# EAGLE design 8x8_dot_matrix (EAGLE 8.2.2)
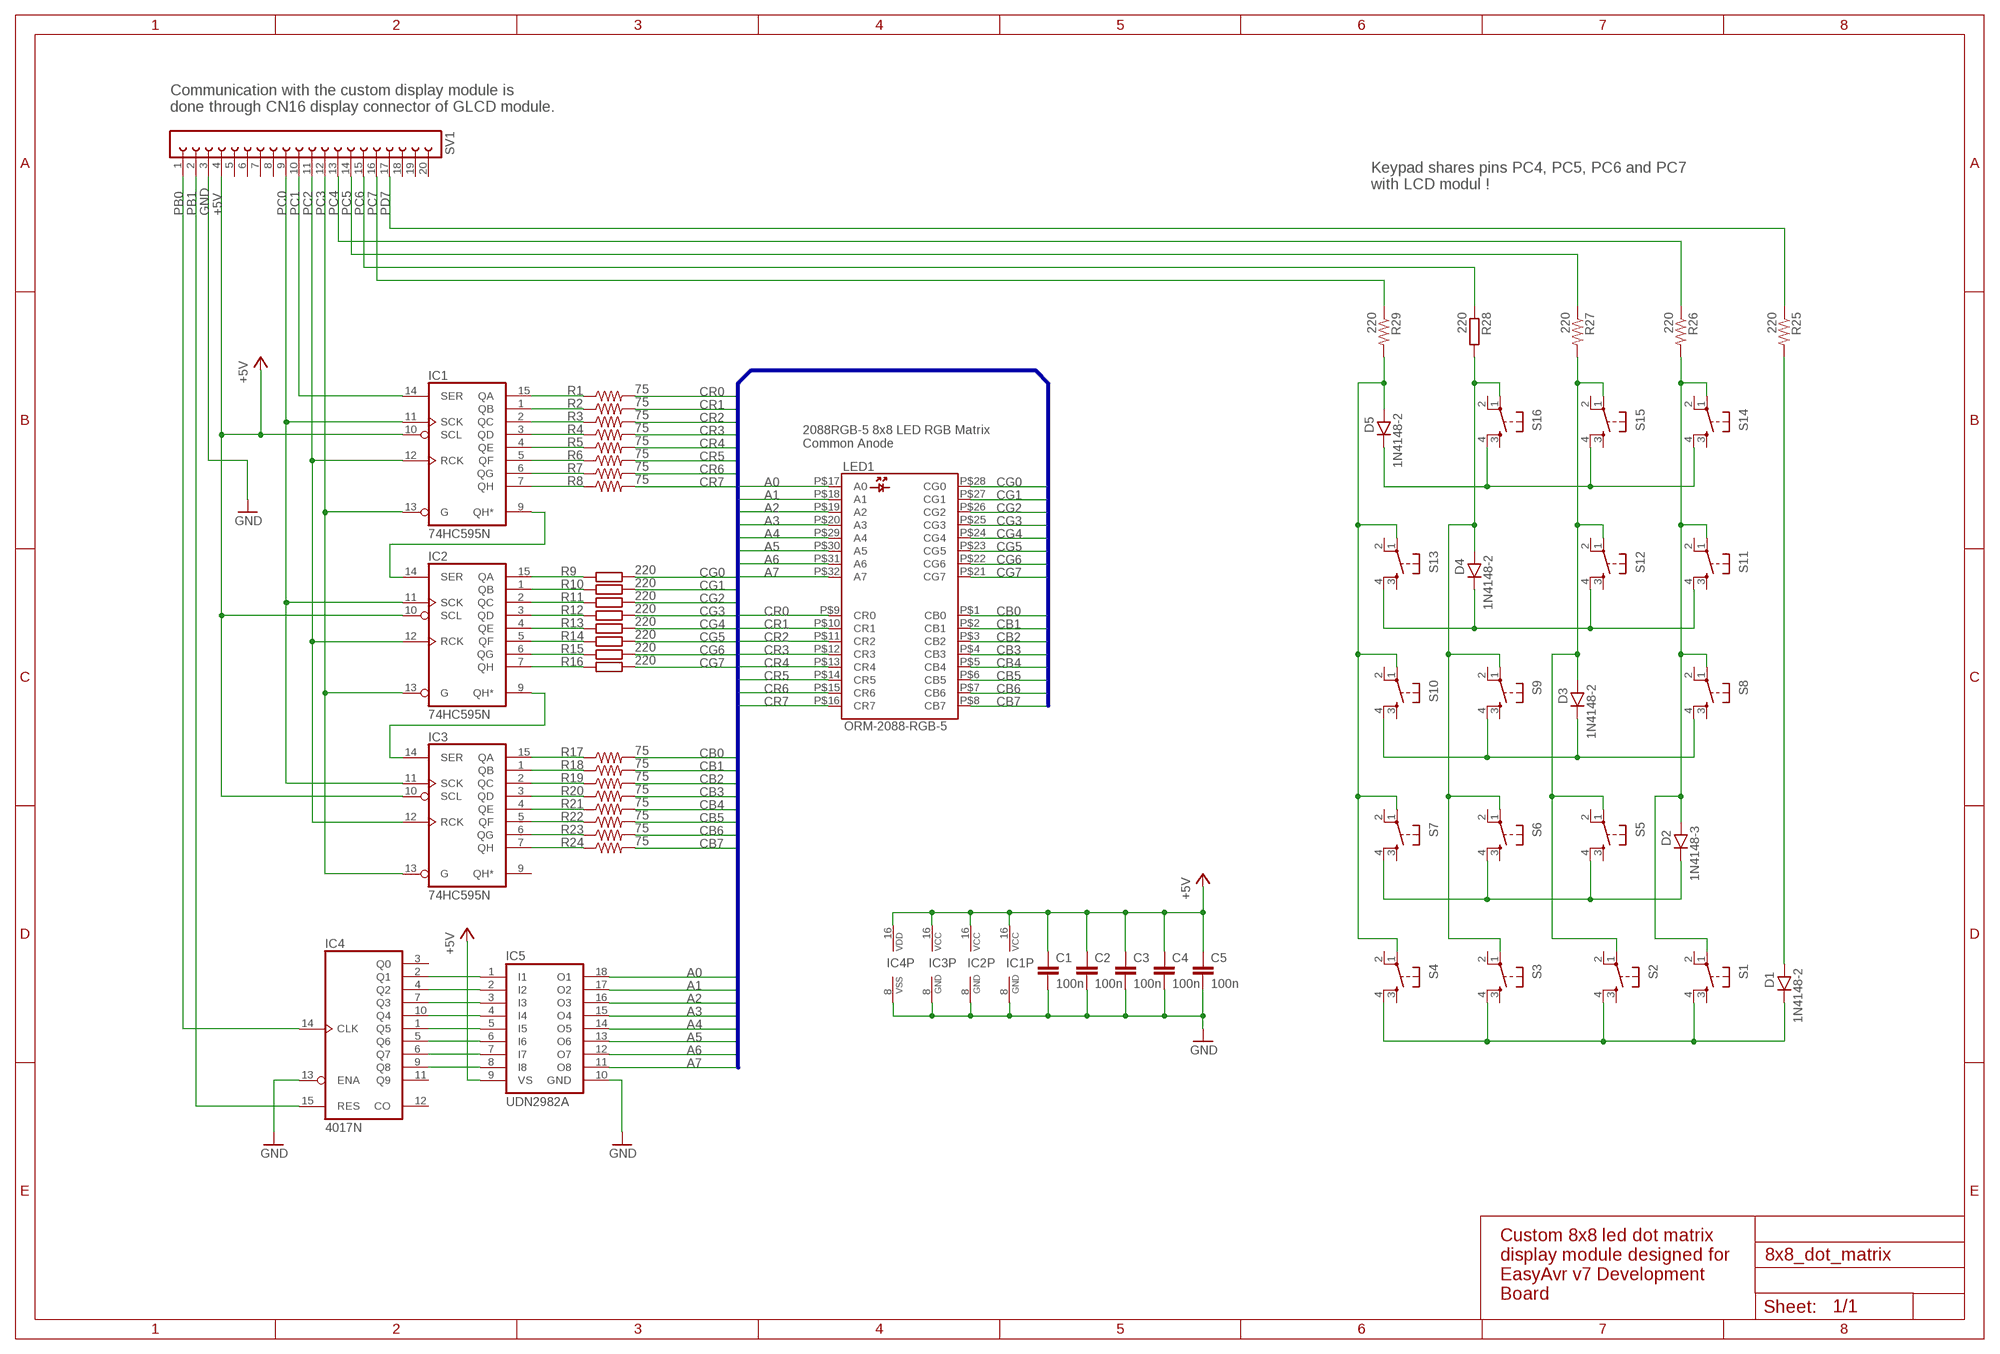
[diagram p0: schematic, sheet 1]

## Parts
C1  100n  C-EU050-024X044  [C050-024X044]
C2  100n  C-EU050-024X044  [C050-024X044]
C3  100n  C-EU050-024X044  [C050-024X044]
C4  100n  C-EU050-024X044  [C050-024X044]
C5  100n  C-EUC0805  [C0805]
D1  1N4148-2  [DO35-2]
D2  1N4148-3  [DO35-3]
D3  1N4148-2  [DO35-2]
D4  1N4148-2  [DO35-2]
D5  1N4148-2  [DO35-2]
IC1  74HC595N  [DIL16]
IC2  74HC595N  [DIL16]
IC3  74HC595N  [DIL16]
IC4  4017N  [DIL16]
IC5  UDN2982A  [DIL18]
LED1  ORM-2088-RGB-5  [ORM-2088-RGB-5]
R1  75  7MM  [0703]
R2  75  7MM  [0703]
R3  75  7MM  [0703]
R4  75  7MM  [0703]
R5  75  7MM  [0703]
R6  75  7MM  [0703]
R7  75  7MM  [0703]
R8  75  7MM  [0703]
R9  220  R-EU_0204/5  [0204/5]
R10  220  R-EU_0204/5  [0204/5]
R11  220  R-EU_0204/5  [0204/5]
R12  220  R-EU_0204/5  [0204/5]
R13  220  R-EU_0204/5  [0204/5]
R14  220  R-EU_0204/5  [0204/5]
R15  220  R-EU_0204/5  [0204/5]
R16  220  R-EU_0204/5  [0204/5]
R17  75  7MM  [0703]
R18  75  7MM  [0703]
R19  75  7MM  [0703]
R20  75  7MM  [0703]
R21  75  7MM  [0703]
R22  75  7MM  [0703]
R23  75  7MM  [0703]
R24  75  7MM  [0703]
R25  220  7MM  [0703]
R26  220  7MM  [0703]
R27  220  7MM  [0703]
R28  220  R-EU_0207/10  [0207/10]
R29  220  7MM  [0703]
S1  DTSM-6  [DTSM-6]
S2  DTSM-6  [DTSM-6]
S3  DTSM-6  [DTSM-6]
S4  DTSM-6  [DTSM-6]
S5  DTSM-6  [DTSM-6]
S6  DTSM-6  [DTSM-6]
S7  DTSM-6  [DTSM-6]
S8  DTSM-6  [DTSM-6]
S9  DTSM-6  [DTSM-6]
S10  DTSM-6  [DTSM-6]
S11  DTSM-6  [DTSM-6]
S12  DTSM-6  [DTSM-6]
S13  DTSM-6  [DTSM-6]
S14  DTSM-6  [DTSM-6]
S15  DTSM-6  [DTSM-6]
S16  DTSM-6  [DTSM-6]
SV1  FE20-1  [FE20]

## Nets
+5V: C1.1 C2.1 C3.1 C4.1 C5.1 IC1.10(SCL) IC1.16(VCC) IC2.10(SCL) IC2.16(VCC) IC3.10(SCL) IC3.16(VCC) IC4.16(VDD) IC5.9(VS) SV1.4
A0: IC5.18(O1) LED1.P$17(A0)
A1: IC5.17(O2) LED1.P$18(A1)
A2: IC5.16(O3) LED1.P$19(A2)
A3: IC5.15(O4) LED1.P$20(A3)
A4: IC5.14(O5) LED1.P$29(A4)
A5: IC5.13(O6) LED1.P$30(A5)
A6: IC5.12(O7) LED1.P$31(A6)
A7: IC5.11(O8) LED1.P$32(A7)
CB0: LED1.P$1(CB0) R17.2
CB1: LED1.P$2(CB1) R18.2
CB2: LED1.P$3(CB2) R19.2
CB3: LED1.P$4(CB3) R20.2
CB4: LED1.P$5(CB4) R21.2
CB5: LED1.P$6(CB5) R22.2
CB6: LED1.P$7(CB6) R23.2
CB7: LED1.P$8(CB7) R24.2
CG0: LED1.P$28(CG0) R9.2
CG1: LED1.P$27(CG1) R10.2
CG2: LED1.P$26(CG2) R11.2
CG3: LED1.P$25(CG3) R12.2
CG4: LED1.P$24(CG4) R13.2
CG5: LED1.P$23(CG5) R14.2
CG6: LED1.P$22(CG6) R15.2
CG7: LED1.P$21(CG7) R16.2
CR0: LED1.P$9(CR0) R1.2
CR1: LED1.P$10(CR1) R2.2
CR2: LED1.P$11(CR2) R3.2
CR3: LED1.P$12(CR3) R4.2
CR4: LED1.P$13(CR4) R5.2
CR5: LED1.P$14(CR5) R6.2
CR6: LED1.P$15(CR6) R7.2
CR7: LED1.P$16(CR7) R8.2
GND: C1.2 C2.2 C3.2 C4.2 C5.2 IC1.8(GND) IC2.8(GND) IC3.8(GND) IC4.8(VSS) IC4.13(ENA) IC5.10(GND) SV1.3
N$1: IC4.2(Q1) IC5.1(I1)
N$2: IC4.4(Q2) IC5.2(I2)
N$3: IC4.7(Q3) IC5.3(I3)
N$4: IC4.10(Q4) IC5.4(I4)
N$5: IC4.1(Q5) IC5.5(I5)
N$6: IC4.5(Q6) IC5.6(I6)
N$7: IC4.6(Q7) IC5.7(I7)
N$8: IC4.9(Q8) IC5.8(I8)
N$9: IC1.9(QH*) IC2.14(SER)
N$10: IC2.9(QH*) IC3.14(SER)
N$11: IC3.7(QH) R24.1
N$12: IC3.6(QG) R23.1
N$13: IC3.5(QF) R22.1
N$14: IC3.4(QE) R21.1
N$15: IC3.3(QD) R20.1
N$16: IC3.2(QC) R19.1
N$17: IC3.1(QB) R18.1
N$18: IC3.15(QA) R17.1
N$19: IC2.7(QH) R16.1
N$20: IC2.6(QG) R15.1
N$21: IC2.5(QF) R14.1
N$22: IC2.4(QE) R13.1
N$23: IC2.3(QD) R12.1
N$24: IC2.2(QC) R11.1
N$25: IC2.1(QB) R10.1
N$26: IC2.15(QA) R9.1
N$27: IC1.7(QH) R8.1
N$28: IC1.6(QG) R7.1
N$29: IC1.5(QF) R6.1
N$30: IC1.4(QE) R5.1
N$31: IC1.3(QD) R4.1
N$32: IC1.2(QC) R3.1
N$33: IC1.1(QB) R2.1
N$34: IC1.15(QA) R1.1
N$35: D2.C S5.4 S6.4 S7.4
N$36: D1.C S1.4 S2.4 S3.4 S4.4
N$37: D1.A R25.2
N$38: D3.C S8.4 S9.4 S10.4
N$39: D4.C S11.4 S12.4 S13.4
N$40: D5.C S14.4 S15.4 S16.4
N$41: D2.A R26.2 S1.1 S8.1 S11.1 S14.1
N$42: D3.A R27.2 S2.1 S5.1 S12.1 S15.1
N$43: D4.A R28.2 S3.1 S6.1 S9.1 S16.1
N$44: D5.A R29.2 S4.1 S7.1 S10.1 S13.1
PB0: IC4.14(CLK) SV1.1
PB1: IC4.15(RES) SV1.2
PC0: IC1.11(SCK) IC2.11(SCK) IC3.11(SCK) SV1.9
PC1: IC1.14(SER) SV1.10
PC2: IC1.12(RCK) IC2.12(RCK) IC3.12(RCK) SV1.11
PC3: IC1.13(G) IC2.13(G) IC3.13(G) SV1.12
PC4: R26.1 SV1.13
PC5: R27.1 SV1.14
PC6: R28.1 SV1.15
PC7: R29.1 SV1.16
PD7: R25.1 SV1.17
Unconnected: IC3.9(QH*) IC4.3(Q0) IC4.11(Q9) IC4.12(CO) S1.2 S1.3 S2.2 S2.3 S3.2 S3.3 S4.2 S4.3 S5.2 S5.3 S6.2 S6.3 S7.2 S7.3 S8.2 S8.3 S9.2 S9.3 S10.2 S10.3 S11.2 S11.3 S12.2 S12.3 S13.2 S13.3 S14.2 S14.3 S15.2 S15.3 S16.2 S16.3 SV1.5 SV1.6 SV1.7 SV1.8 SV1.18 SV1.19 SV1.20

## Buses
A[0..7],CR[0..7],CG[0..7],CB[0..7]

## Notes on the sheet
- Communication with the custom display module is
  done through CN16 display connector of GLCD module.
- Keypad shares pins PC4, PC5, PC6 and PC7
  with LCD modul !
- 2088RGB-5 8x8 LED RGB Matrix 
  Common Anode
- Custom 8x8 led dot matrix 
  display module designed for
  EasyAvr v7 Development
  Board

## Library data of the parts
C1-C5 = rcl:C-EU: CAPACITOR, European symbol
D1-D5 = gm-diodes:1N4148: Fast Switching Diode
IC1-IC3 = 74xx-eu:74*595: 8-bit SHIFT REGISTER, output latch
IC4 = 40xx:4017: COUNTER/DIVIDER
IC5 = uln-udn:UDN298*: DRIVER ARRAY Source: Allegro Microsystems Inc. / UDN2981-UDN2984.pdf
LED1 = LED:ORM-2088-RGB-5: ORM 2088RGB-5 8x8 LED RGB Matrix
R1-R8 R17-R27 R29 = gm-resistors:7MM: 7mm Resistors
R9-R16 R28 = rcl:R-EU_: RESISTOR, European symbol
S1-S16 = switch-tact:DTSM-6
SV1 = con-lsta:FE20-1: FEMALE HEADER; OC_FARNELL: unknown; OC_NEWARK: unknown

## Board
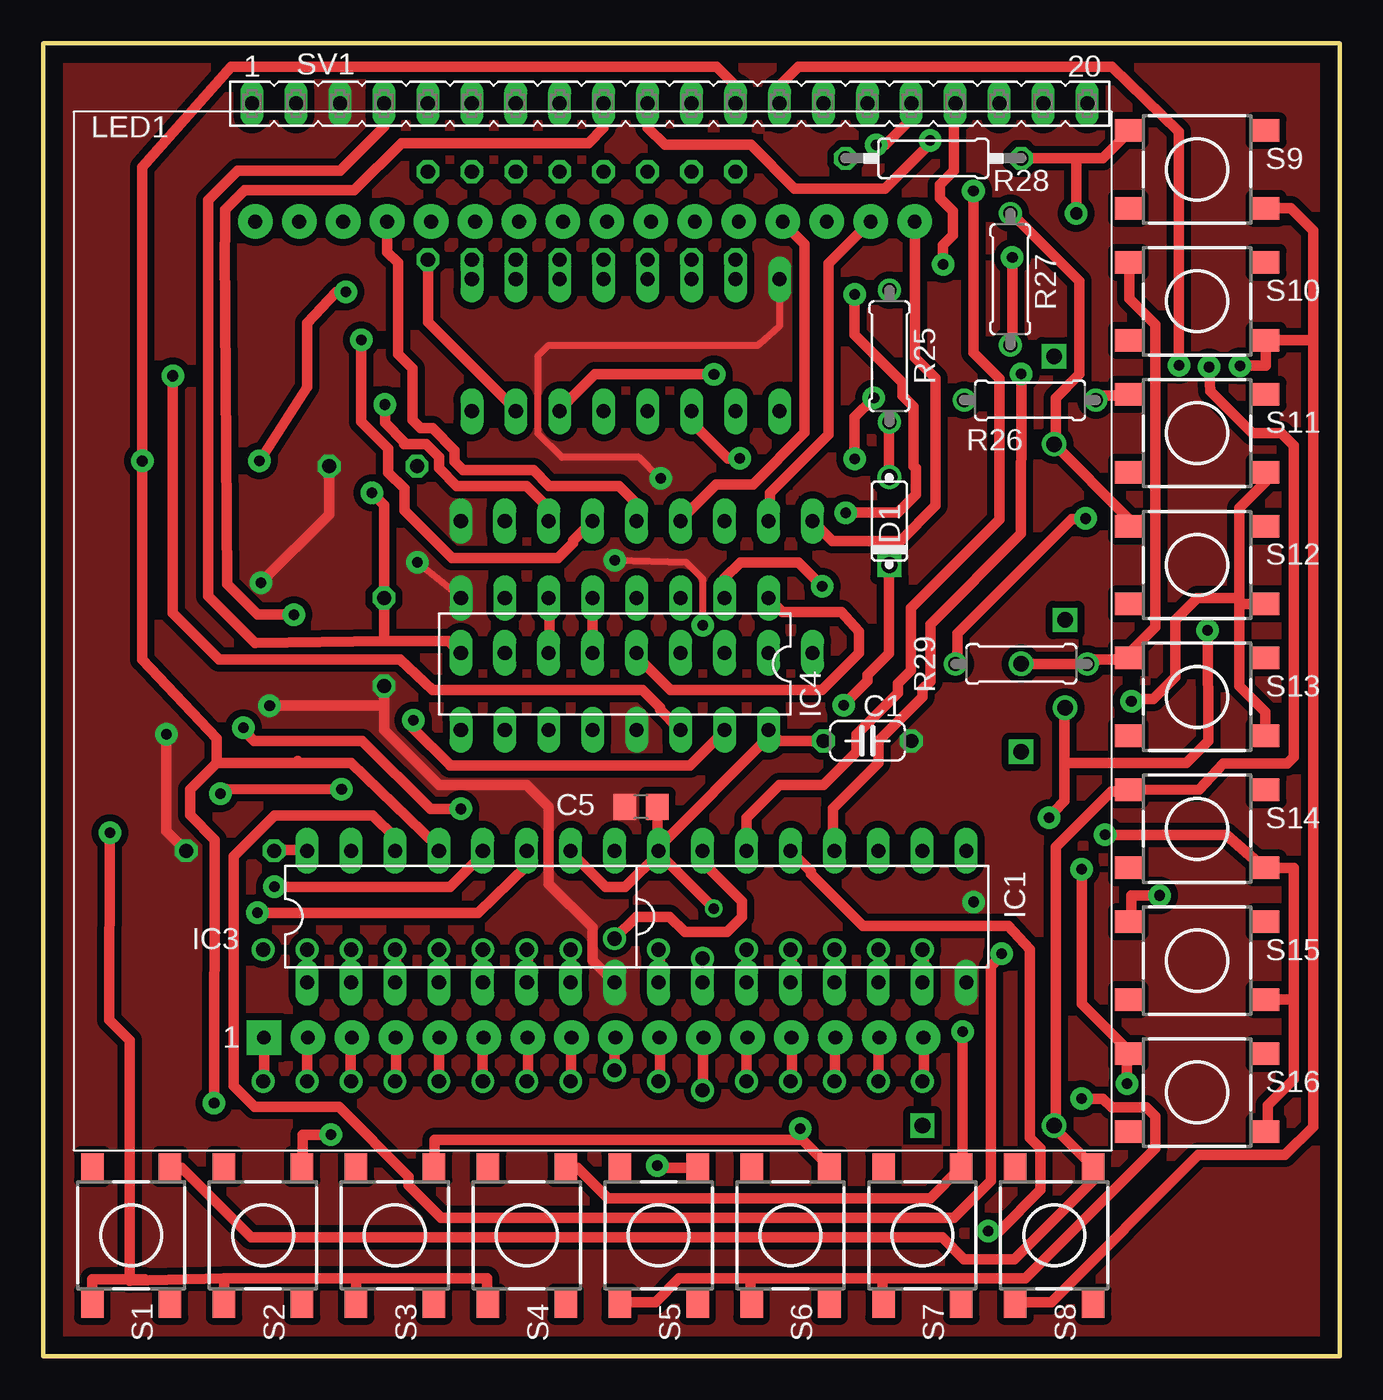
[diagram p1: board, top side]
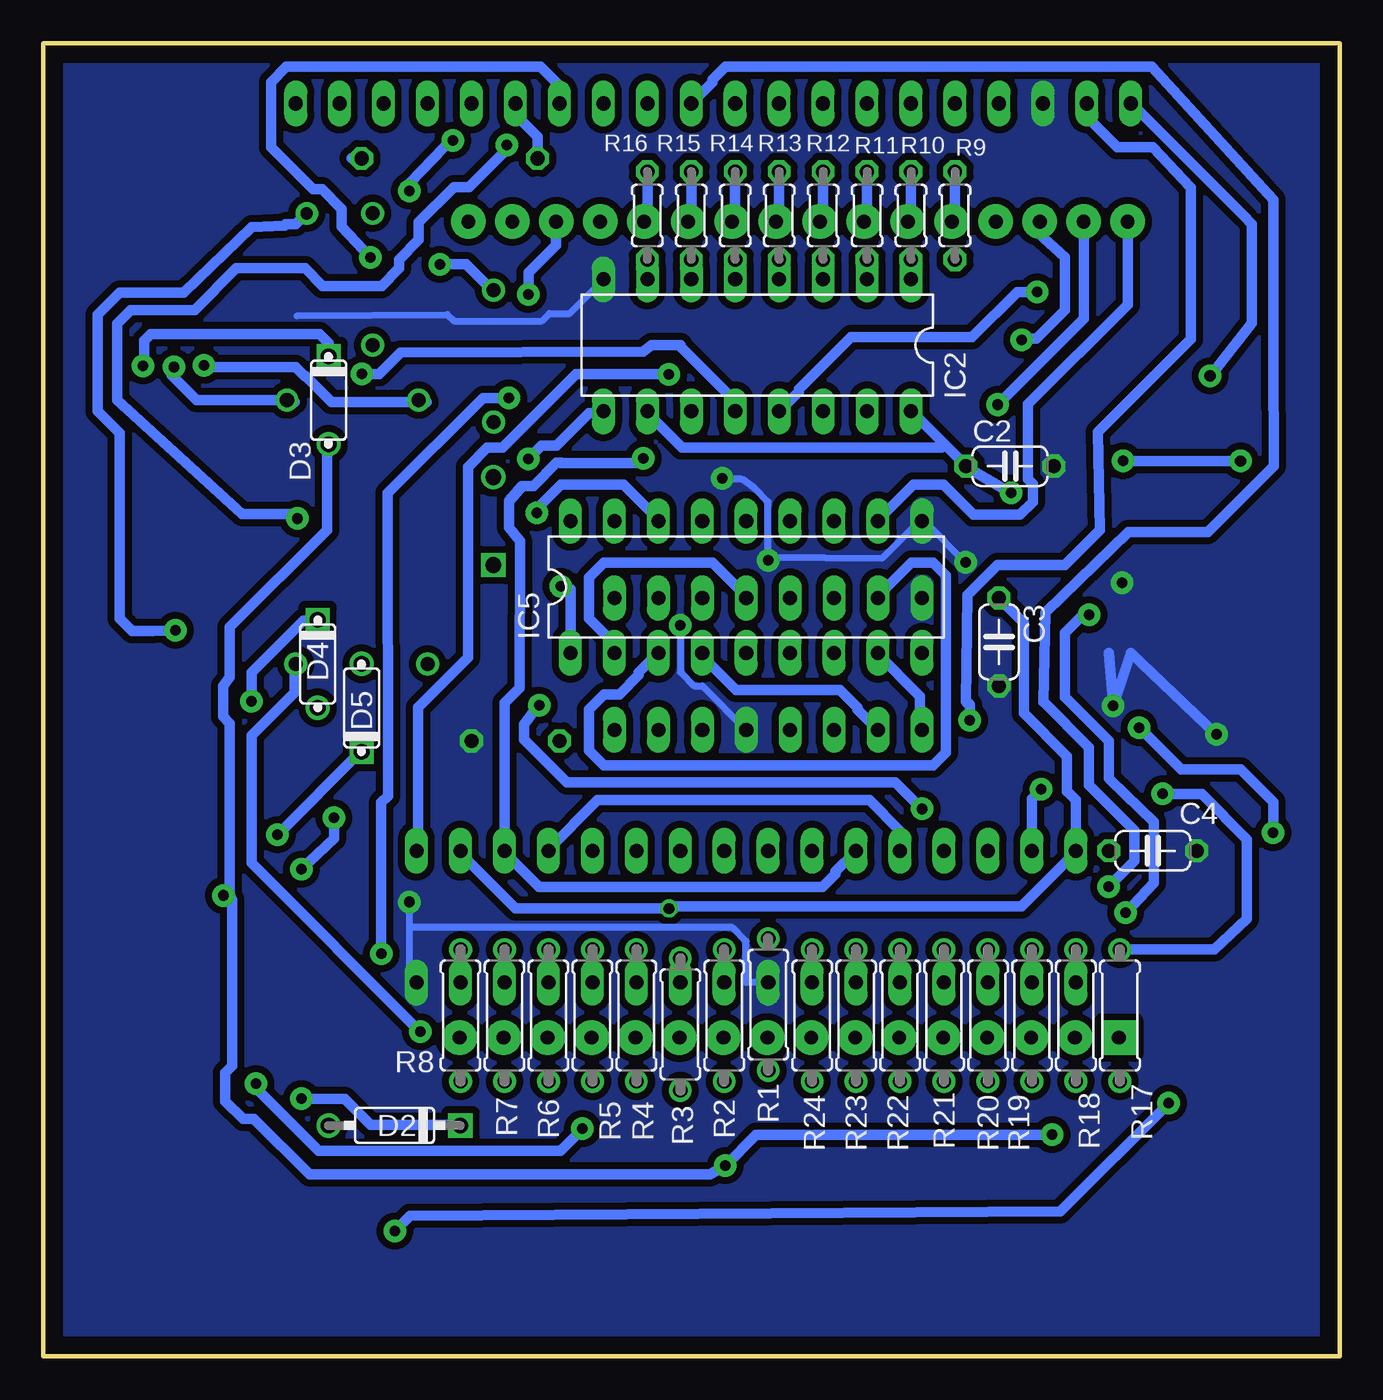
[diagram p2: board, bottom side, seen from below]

Size 74.91 x 75.87 mm. Coordinates in mm from the lower left corner, seen from the top.
Outline: 0,0 74.91,0 74.91,75.87 0,75.87 0,0
Copper layers (1*16): Top 0.035mm / dielectric 1.5mm / Bottom 0.035mm
Design rules "default *": minimum track width 16mil, minimum drill 24mil, track to track 12mil, track to pad 12mil, pad to pad 12mil, via to via 12mil, smd to smd 12mil, copper to edge 40mil, drill to drill 12mil, minimum pad ring 10mil, minimum via ring 8mil, stop-mask expansion 4mil, vias tented up to drill 0mil, thermal gap 10mil

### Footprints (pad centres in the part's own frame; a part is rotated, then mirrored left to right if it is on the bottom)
C050-024X044 = drill 0.813 octagon: 1 -2.54,0; 2 2.54,0
C0805 = smd 1.3 x 1.5: 1 -0.95,0; 2 0.95,0
DO35-2 = drill 0.9: A 2.54,0 | drill 0.9 square: C -2.54,0
DO35-3 = drill 0.9: A 3.81,0 | drill 0.9 square: C -3.81,0
DIL16 = drill 0.813 long: 1 -8.89,-3.81; 2 -6.35,-3.81; 3 -3.81,-3.81; 4 -1.27,-3.81; 5 1.27,-3.81; 6 3.81,-3.81; 7 6.35,-3.81; 8 8.89,-3.81; 9 8.89,3.81; 10 6.35,3.81; 11 3.81,3.81; 12 1.27,3.81; 13 -1.27,3.81; 14 -3.81,3.81; 15 -6.35,3.81; 16 -8.89,3.81
DIL18 = drill 0.813 long: 1 -10.16,-3.81; 2 -7.62,-3.81; 3 -5.08,-3.81; 4 -2.54,-3.81; 5 0,-3.81; 6 2.54,-3.81; 7 5.08,-3.81; 8 7.62,-3.81; 9 10.16,-3.81; 10 10.16,3.81; 11 7.62,3.81; 12 5.08,3.81; 13 2.54,3.81; 14 0,3.81; 15 -2.54,3.81; 16 -5.08,3.81; 17 -7.62,3.81; 18 -10.16,3.81
ORM-2088-RGB-5 = drill 0.8 pad 2 square: P$1 -19,-23.5 | drill 0.8 pad 2: P$2 -16.46,-23.5; P$3 -13.92,-23.5; P$4 -11.38,-23.5; P$5 -8.84,-23.5; P$6 -6.3,-23.5; P$7 -3.76,-23.5; P$8 -1.22,-23.5; P$9 1.32,-23.5; P$10 3.86,-23.5; P$11 6.4,-23.5; P$12 8.94,-23.5; P$13 11.48,-23.5; P$14 14.02,-23.5; P$15 16.56,-23.5; P$16 19.1,-23.5; P$17 18.6,23.66; P$18 16.06,23.66; P$19 13.52,23.66; P$20 10.98,23.66; P$21 8.44,23.66; P$22 5.9,23.66; P$23 3.36,23.66; P$24 0.82,23.66; P$25 -1.72,23.66; P$26 -4.26,23.66; P$27 -6.8,23.66; P$28 -9.34,23.66; P$29 -11.88,23.66; P$30 -14.42,23.66; P$31 -16.96,23.66; P$32 -19.5,23.66
0703 = drill 0.813: 1 -3.81,0; 2 3.81,0
0204/5 = drill 0.813 octagon: 1 -2.54,0; 2 2.54,0
0207/10 = drill 0.813 octagon: 1 -5.08,0; 2 5.08,0
DTSM-6 = smd 1.55 x 1.3: 1 -3.975,2.25; 2 3.975,2.25; 3 -3.975,-2.25; 4 3.975,-2.25
FE20 = drill 0.813 long: 1 -24.13,0; 2 -21.59,0; 3 -19.05,0; 4 -16.51,0; 5 -13.97,0; 6 -11.43,0; 7 -8.89,0; 8 -6.35,0; 9 -3.81,0; 10 -1.27,0; 11 1.27,0; 12 3.81,0; 13 6.35,0; 14 8.89,0; 15 11.43,0; 16 13.97,0; 17 16.51,0; 18 19.05,0; 19 21.59,0; 20 24.13,0

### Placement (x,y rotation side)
C1  47.62,35.56 0 top
C2  19.05,51.44 0 bottom
C3  19.68,41.27 270 bottom
C4  10.79,29.21 0 bottom
C5  34.54,31.75 180 top
D1  48.9,48.26 90 top
D2  54.61,13.34 180 bottom
D3  58.42,55.24 270 bottom
D4  59.05,40.01 270 bottom
D5  56.52,37.47 90 bottom
IC1  44.45,25.4 0 top
IC2  33.66,58.42 180 bottom
IC3  24.13,25.4 0 top
IC4  33.02,40.01 180 top
IC5  34.29,44.45 0 bottom
LED1  31.75,41.91 0 top
R1  33.02,20.32 270 bottom
R2  35.56,19.68 270 bottom
R3  38.1,19.18 270 bottom
R4  40.64,19.68 270 bottom
R5  43.18,19.68 270 bottom
R6  45.72,19.68 270 bottom
R7  48.26,19.68 270 bottom
R8  50.8,19.68 270 bottom
R9  22.23,65.91 90 bottom
R10  24.77,65.91 90 bottom
R11  27.3,65.91 90 bottom
R12  29.84,65.91 90 bottom
R13  32.38,65.91 90 bottom
R14  34.92,65.91 90 bottom
R15  37.47,65.91 90 bottom
R16  40.01,65.91 90 bottom
R17  12.7,19.68 270 bottom
R18  15.24,19.68 270 bottom
R19  17.78,19.68 270 bottom
R20  20.32,19.68 270 bottom
R21  22.86,19.68 270 bottom
R22  25.4,19.68 270 bottom
R23  27.94,19.68 270 bottom
R24  30.48,19.68 270 bottom
R25  48.9,57.78 270 top
R26  57.02,55.24 0 top
R27  55.88,62.23 90 top
R28  51.44,69.22 0 top
R29  56.52,40.01 0 top
S1  5.08,6.99 270 top
S2  12.7,6.99 270 top
S3  20.32,6.99 270 top
S4  27.94,6.99 270 top
S5  35.56,6.99 270 top
S6  43.18,6.99 270 top
S7  50.8,6.99 270 top
S8  58.42,6.99 270 top
S9  66.67,68.58 0 top
S10  66.67,60.96 0 top
S11  66.67,53.34 0 top
S12  66.67,45.72 0 top
S13  66.67,38.1 0 top
S14  66.67,30.48 0 top
S15  66.67,22.86 0 top
S16  66.67,15.24 0 top
SV1  36.2,72.39 0 top

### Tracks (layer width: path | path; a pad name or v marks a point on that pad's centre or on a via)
+5V  (via drill 0.61, 0.61 pad 1.3)
  Top 0.61: IC3.10 30.5,29.12 32.5,27.12 33.62,27.12 35.62,29.12 IC1.16 | 35.62,29.5 41.88,35.75 41.88,36.12 IC4.16 42.55,35.56 C1.1 | 35.62,29.5 IC1.16 | v38.75,25.88 35.75,28.88 IC1.16 | C4.1 13.38,29.25 15.12,29.25 IC3.16 | 19.62,72.38 SV1.4 19.68,71.04 17.14,68.5 11.22,68.5 9.53,66.8 9.53,43.94 12.25,41.22 19.83,41.34 | 18.99,49.84 v18.99,49.88 19.68,49.19 C3.1 19.68,41.49 19.83,41.34 | IC5.9 23.43,41.34 19.83,41.34 | 35.56,29.57 35.62,29.5 | C5.1 35.49,29.28 IC1.16
  Bottom 0.61: 50.75,29.12 IC1.10 | 22.81,52.69 24.75,54.62 IC2.16 | 22.81,52.69 21.62,51.5 C2.1 21.38,51.25 v18.99,49.88 | IC2.10 40,54.5 38,52.5 23,52.5 22.81,52.69 | C3.1 19.62,43.75 18.25,42.38 18.25,37.16 18.24,37.16 15.75,34.67 15.75,32.64 15.62,32.51 15.25,32.13 15.25,29.25 IC3.16 15.38,29 18.38,26 38.5,26 v38.75,25.88 47.62,25.88 50.75,29 50.75,29.12 | 50.8,29.18 50.75,29.12 | 35.56,29.84 IC1.16
A0
  Top 0.61: 44.49,48.25 44.5,48.25 IC5.18 45.59,47.12 49.53,47.12 51.56,49.15 51.56,56.52 50.38,57.7 50.38,65.5 LED1.P$17
A1
  Top 0.61: IC5.17 42,48.38 42,49.88 45.38,53.25 45.38,63.12 47.75,65.5 LED1.P$18
A2  (via drill 0.61 pad 1.3)
  Top 0.61: v46.88,61.37 46.88,59.04 49.66,56.26 49.66,55.5 50.29,54.86 50.29,51.44 50.42,51.31 50.42,49.78 49.38,48.75 v46.38,48.75
  Bottom 0.61: v46.38,48.75 46.38,49 45,50.38 41.38,50.38 39.38,48.38 IC5.16 | LED1.P$19 45.27,64.2 46.86,62.61 46.86,61.38 v46.88,61.37
A3
  Top 0.61: IC5.15 36.88,48.38 38.88,50.38 41,50.38 44,53.38 44,64.25 42.75,65.5 LED1.P$20
A4
  Top 0.61: LED1.P$29 19.88,65.5 19.88,63.8 20.49,63.18 20.49,57.91 21.34,57.06 21.34,54.1 21.82,53.62 22.5,53.62 23.77,52.34 23.77,51.69 24.26,51.21 28.32,51.21 29.23,50.29 33.27,50.29 34.29,49.28 IC5.14
A5  (via drill 0.61 pad 1.3)
  Top 0.61: v18.38,58.73 18.38,54.02 19.94,52.45 19.94,51.05 20.87,50.12 20.88,50.12 20.88,48.88 23.62,46.12 29.75,46.12 30.62,47 30.62,47.12 IC5.13
  Bottom 0.61: LED1.P$30 17.38,65.5 17.38,64.87 15.88,63.5 15.88,60.45 17.53,58.8 18.3,58.8 v18.38,58.73
A6  (via drill 0.61 pad 1.3)
  Top 0.61: v19.75,54.99 19.75,53.94 20.85,52.83 20.85,52.7 21.06,52.7 22.12,52.7 22.86,51.96 22.86,51.31 23.88,50.29 27.94,50.29 29.21,49.02 IC5.12
  Bottom 0.61: v19.75,54.99 19.62,55.09 | v19.75,54.99 19.62,55.12 | LED1.P$31 14.79,59.95 v19.75,54.99
A7
  Bottom 0.61: 22.91,50.38 22.88,50.38 | 22.91,50.38 24.62,50.38 26.62,48.38 IC5.11 | 22.91,50.38 21.17,48.64 19.53,48.64 19.51,48.62 18.47,48.62 17.73,49.36 17.73,50.4 18,50.67 18,55.02 12.25,60.77 LED1.P$32
CB0
  Top 0.61: LED1.P$1 12.75,15.88 R17.2
CB1
  Top 0.61: R18.2 15.25,18.38 LED1.P$2
CB2
  Top 0.61: R19.2 17.75,15.88 17.75,18.38 LED1.P$3
CB3
  Top 0.61: R20.2 20.38,15.88 20.38,18.38 LED1.P$4
CB4
  Top 0.61: R21.2 22.88,15.88 22.88,18.38 LED1.P$5
CB5
  Top 0.61: R22.2 25.38,15.88 25.38,18.38 LED1.P$6
CB6
  Top 0.61: R23.2 28,15.88 28,18.38 LED1.P$7
CB7
  Top 0.61: R24.2 30.5,15.88 30.5,18.38 LED1.P$8
CG0
  Bottom 0.61: R9.2 22.23,65.75 LED1.P$28
CG1
  Bottom 0.61: R10.2 24.77,65.75 LED1.P$27
CG2
  Bottom 0.61: R11.2 27.3,65.75 LED1.P$26
CG3
  Bottom 0.61: R12.2 29.84,65.75 LED1.P$25
CG4
  Bottom 0.61: R13.2 32.38,65.75 LED1.P$24
CG5
  Bottom 0.61: R14.2 34.92,65.75 LED1.P$23
CG6
  Bottom 0.61: R15.2 37.47,65.75 LED1.P$22
CG7
  Bottom 0.61: R16.2 40.01,65.75 LED1.P$21
CR0
  Top 0.61: R1.2 33,16.51 33,18.38 LED1.P$9
CR1
  Top 0.61: R2.2 35.62,15.88 35.62,18.38 LED1.P$10
CR2
  Top 0.61: R3.2 38.12,15.88 38.12,18.38 LED1.P$11
CR3
  Top 0.61: R4.2 40.62,15.88 40.62,18.38 LED1.P$12
CR4
  Top 0.61: R5.2 43.25,15.88 43.25,18.38 LED1.P$13
CR5
  Top 0.61: R6.2 45.75,15.88 45.75,18.38 LED1.P$14
CR6
  Top 0.61: R7.2 48.25,18.38 LED1.P$15
CR7
  Top 0.61: R8.2 50.88,15.88 50.88,18.38 LED1.P$16
GND  (via drill 0.61 pad 1.3)
  Top 0.406: v21.62,45.87 24.12,43.88 IC4.8 | v38.1,42.23 38.1,44.93 37.15,45.88 v33.02,46.01 | IC2.8 42.55,59.53 41.4,58.52 41.27,58.42 29.21,58.42 28.57,57.78 28.57,53.34 29.97,51.94 34.42,51.94 35.56,50.8 v35.69,50.74
  Top 0.61: IC3.8 31.75,22.86 31.75,24.77 29.21,27.3 29.21,31.75 27.94,33.02 22.86,33.02 19.68,36.2 C3.2 19.68,37.59 v13.08,37.59 | C4.2 7.11,30.35 v7.11,35.94 | C2.2 16.51,48.64 v12.57,44.7
  Bottom 0.406: 53.75,24.77 53.75,21.62 53.38,21.62 IC1.8 | 53.75,24.77 v53.75,26.25 | 60.26,60.12 51.56,60.2 51.18,59.82 46.1,59.82 45.67,60.25 44.5,60.25 42.62,62.12 IC2.8 | v21.62,45.87 24,48.25 IC5.10 24.29,48.26 26.45,46.1 33,46.15 | 53.75,24.77 35.08,24.77 34.29,23.97 34.29,21.59 IC3.8 | IC4.13 36.83,38.73 37.31,38.73 38.1,39.53 v38.1,42.23 | 33,46.15 v33.02,46.01 | v35.69,50.74 35.75,50.67 34.54,50.67 33.81,50.16 33.02,49.37 33.02,46.35 33.08,45.97 33,46.15
  Bottom 0.61: v7.11,35.94 12.06,40.64 v13.08,37.59 13.34,40.64
  pour Bottom (isolate 0.406, no thermals): 0,0 74.93,0 74.93,75.56 0,75.56
  pour Top (isolate 0.406, no thermals): 0,75.56 74.93,75.56 74.93,0 0,0
N$1  (via drill 0.61 pad 1.3)
  Top 0.61: v45.01,44.5 43.63,45.88 40.29,45.88 39.37,44.96 IC4.2
  Bottom 0.61: v45.01,44.5 44.45,44.33 IC5.1
N$2
  Bottom 0.61: IC5.2 42,40.75 42,41.25 43.38,42.62 43.38,45 42.5,45.88 36.25,45.88 34.25,43.88 IC4.4
N$3
  Bottom 0.61: IC5.3 39.38,40.62 40.5,39.5 40.5,39.38 41.62,38.25 42.5,38.25 43.38,37.38 43.38,35 42.5,34.12 23.5,34.12 22.75,34.88 22.75,45.12 23.5,45.88 24.75,45.88 26.75,43.88 IC4.7
N$4
  Bottom 0.61: IC4.10 26.75,36.25 27.88,37.38 27.88,37.5 28.88,38.5 34.88,38.5 36.75,40.38 36.75,40.62 IC5.4
N$5
  Top 0.61: IC5.5 34.38,40.62 34.38,40.38 36.25,38.5 45,38.5 47.12,40.62 47.12,41.88 46.13,43 42.73,43 IC4.1
N$6
  Top 0.61: IC4.5 IC5.6
N$7
  Top 0.61: IC5.7 29.25,40.75 29.25,43.75 IC4.6
N$8
  Bottom 0.61: IC4.9 24.25,36.25 24.25,38.12 26.75,40.62 IC5.8
N$9  (via drill 0.61 pad 1.3)
  Top 0.61: v38.76,56.75 31.88,56.75 29.75,54.62 IC2.14
  Bottom 0.61: v38.76,56.75 44.12,56.75 48.38,52.5 49.25,52.5 50.38,51.38 50.38,40.38 53.25,37.5 53.25,29.25 IC1.9
N$10  (via drill 0.61 pad 1.3)
  Top 0.61: v55.38,23.26 54.75,22.51 54.75,10.12 52.62,8 23,8 21.12,9.88 21.12,10.38 17.09,14.4 12.22,14.4 11,15.62 11,28.88 13.38,31.25 19.04,31.25 20.32,29.97 IC3.14 | v48,55.38 46.88,54.26 v46.88,51.86
  Bottom 0.61: v55.38,23.26 55.38,32 54.99,32.38 55,49.88 49.5,55.38 v48,55.38 | IC2.9 42.62,54.5 43.38,54.5 45.25,52.62 46.12,52.62 v46.88,51.86
N$11
  Top 0.61: IC3.7 30.5,21.62 30.5,23.38 R24.1
N$12
  Top 0.61: IC3.6 28,21.62 28,23.38 R23.1
N$13
  Top 0.61: IC3.5 25.38,21.62 25.38,23.38 R22.1
N$14
  Top 0.61: IC3.4 22.88,21.62 22.88,23.38 R21.1
N$15
  Top 0.61: IC3.3 20.38,21.62 20.38,23.38 R20.1
N$16
  Top 0.61: IC3.2 17.75,21.62 17.75,23.38 R19.1
N$17
  Top 0.61: IC3.1 15.25,21.62 15.25,23.38 R18.1
N$18  (via drill 0.61 pad 1.3)
  Top 0.61: v17.24,32.75 10.54,32.77 10.28,32.5 v10.23,32.5
  Bottom 0.61: v10.23,32.5 7.98,32.5 5.35,29.88 5.35,25.26 7.24,23.5 12,23.5 12.62,23.5 R17.1 | IC3.15 17.78,32.21 v17.24,32.75
N$19
  Bottom 0.61: R16.1 IC2.7
N$20
  Bottom 0.61: R15.1 IC2.6
N$21
  Bottom 0.61: R14.1 IC2.5
N$22
  Bottom 0.61: R13.1 IC2.4
N$23
  Bottom 0.61: R12.1 IC2.3
N$24
  Bottom 0.61: R11.1 IC2.2
N$25
  Bottom 0.61: R10.1 IC2.1
N$26
  Top 0.61: IC2.15 27.38,54.62 22.25,59.75 22.25,60.25 22.23,60.27 R9.1
N$27
  Top 0.61: IC1.7 50.88,21.62 50.88,23.38 R8.1
N$28
  Top 0.61: IC1.6 48.25,21.62 48.25,23.38 R7.1
N$29
  Top 0.61: IC1.5 45.75,21.62 45.75,23.38 R6.1
N$30
  Top 0.61: IC1.4 43.25,21.62 43.25,23.38 R5.1
N$31
  Top 0.61: IC1.3 40.62,21.62 40.62,23.38 R4.1
N$32
  Top 0.61: IC1.2 38.12,21.62 38.12,23.38 R3.1
N$33
  Top 0.61: IC1.1 35.62,21.62 35.62,23.38 R2.1
N$34
  Top 0.61: R1.1 34.29,25.4 36.2,25.4 37.08,24.51 39.5,24.51 40.39,25.4 40.39,26.29 38.1,28.57 IC1.15
N$35  (via drill 0.61 pad 1.3)
  Top 0.61: S5.4 33.38,3.12 35.38,3.12 36.75,4.5 40.88,4.5 | S6.4 40.88,3.12 40.88,4.5 | S7.4 48.5,3.12 48.5,4.5 | v60,14.88 61.24,14.88 61.74,14.38 63.75,14.38 64.25,13.88 64.25,12 56.75,4.5 48.5,4.5 | 40.88,4.5 48.5,4.5
  Bottom 0.61: v60,14.88 57.49,14.88 55.99,13.38 50.88,13.38 D2.C
N$36  (via drill 0.61 pad 1.3)
  Top 0.61: 2.88,3.12 S1.4 2.83,4.45 5.88,4.45 4.99,4.37 | 4.99,4.37 10.45,4.5 | 18,3.12 S3.4 18.07,4.5 | 10.45,4.5 18.07,4.5 | 18.07,4.5 25.64,4.5 25.64,3.12 25.62,3.12 S4.4 | v24.12,31.62 22.38,31.62 18.41,35.56 12.19,35.56 11.58,36.17 v11.58,36.33 | 4.99,4.37 4.99,18.25 3.81,19.43 v3.84,30.24 | D1.C 48.88,45.62 48.88,40.62 47.62,39.37 47.62,39.01 v46.24,37.62 | S2.4 10.45,4.5
  Bottom 0.61: v46.24,37.62 46.5,37.38 47.12,36.5 47.12,35.62 44.65,33.15 25.65,33.15 24.13,31.62 v24.12,31.62 | v3.84,30.24 3.84,32.04 5.71,33.91 9.14,33.91 9.4,34.16 v11.58,36.33
N$37
  Top 0.61: R25.2 48.88,53.88 48.88,50.88 D1.A
N$38  (via drill 0.61 pad 1.3)
  Top 0.61: 73.38,58.71 73.38,65.06 72.1,66.33 S9.4 70.75,66.25 | 73.38,58.71 73.38,13.25 71.75,11.62 66.75,11.62 58.25,3.12 56.25,3.12 S8.4 | 70.75,58.62 S10.4 | S10.4 73.38,58.71 | v69.16,57.24 70.65,57.24 S10.4
  Bottom 0.61: v69.16,57.24 69.16,57.46 69.09,57.53 69.09,58.67 68.71,59.05 58.93,59.05 58.42,58.55 D3.C
N$39  (via drill 0.61 pad 1.3)
  Top 0.61: 69.12,43.81 69.12,43.47 | 69.12,43.47 69.12,38.74 70.62,37.24 70.62,35.88 S13.4 | 70.62,43.38 S12.4 69.12,43.47 | 69.12,43.81 69.12,49 70.62,50.5 70.62,51 S11.4 | v62.88,37.86 62.89,37.97 64.14,37.97 65.41,39.24 65.41,42.55 66.67,43.81 69.12,43.81
  Bottom 0.61: v62.88,37.86 62.88,39.5 59.88,42.5 59.12,42.5 D4.C
N$40  (via drill 0.61 pad 1.3)
  Top 0.61: S16.4 70.75,13 70.75,14.49 72.25,15.99 72.25,20.61 | 70.75,20.5 S15.4 72.25,20.61 | 72.25,20.61 72.25,28.23 S14.4 | 70.75,28.12 S14.4 | v61.37,30.13 68.37,30.13 70.38,28.38 S14.4
  Bottom 0.61: v61.37,30.13 56.62,34.88 D5.C
N$41  (via drill 0.61 pad 1.3)
  Top 0.61: S1.1 7.38,10.88 8,10.88 12,6.88 51.94,6.86 53.2,5.61 56.12,5.61 60.75,10.24 S8.1 60.5,11.12 58.5,13.12 D2.A 58.5,13.38 58.5,29.42 61.71,32.62 62.62,32.62 S14.1 66.81,32.75 68.19,34.25 71.88,34.25 72.25,34.62 72.25,52.63 71.55,53.34 69.85,53.34 67.43,55.76 v67.36,57.16 | S11.1 62.62,55.5 61.01,55.5 60.88,55.12 R26.2
  Bottom 0.61: v67.36,57.16 67.49,56.7 66.04,55.24 R26.2 60.38,55.12
N$42  (via drill 0.61 pad 1.3)
  Top 0.61: S2.1 15,10.88 15,12.8 v16.62,12.8 | S5.1 37.75,10.88 35.49,10.88 v35.49,11.01 | v64.51,26.63 62.87,26.63 62.87,25.4 62.75,25.12 S15.1 | S12.1 62.62,48 62.62,48.5 D3.A 58.5,53 58.5,55.38 59.88,56.75 59.88,62.12 56,66 R27.2
  Bottom 0.61: v16.62,12.8 33.72,12.8 v35.49,11.01 36.38,10.5 59.52,10.5 62.74,13.72 63.37,13.72 64.39,14.73 64.39,16.38 64,16.77 64,26.36 | D3.A 58.5,52.62 58.5,47.75 64.12,42.12 64.14,39.24 64.52,38.73 64.52,36.96 64.14,36.58 64.14,26.5 64,26.36 | v64.51,26.63 64.12,26.63 64,26.36
N$43  (via drill 0.61 pad 1.3, 0.7 pad 1.3)
  Top 0.61: S9.1 62.75,70.75 61.22,69.22 59.69,69.22 | 44.12,12.25 45.38,11 S6.1 | 44.12,12.25 43.88,12.5 22.62,12.5 22.62,11 S3.1 | v62.62,15.75 62.62,17.38 S16.1 62.62,17.75 60,20.37 v60,28.14 | 44.12,12.25 43.81,12.57 43.75,12.64 v43.75,13.14 | v58.11,31.13 58.93,32 59,32.08 59,34.22 | 59,34.22 59,37.38 D4.A | v67.28,41.95 67.31,35.56 66.04,34.29 59.07,34.29 59,34.22 | R28.2 59.69,69.22 | 59.69,69.22 v59.69,66.04
  Bottom 0.61: v62.62,15.75 62.62,15.5 59,11.88 45.02,11.88 v43.75,13.14 | v58.11,31.13 58.11,29.91 v60,28.14 | v67.28,41.95 68.58,41.91 69.78,41.91 70.5,42.62 70.5,53.35 71.75,54.61 71.75,60.2 70.48,61.47 66.8,61.47 62.88,65.25 60.97,65.33 60.89,65.41 60.33,65.41 v59.69,66.04 | R28.2 57.08,69.22
N$44  (via drill 0.61 pad 1.3)
  Top 0.61: S4.1 30.25,10.88 30.88,10.88 32.62,9.12 51.25,9.12 53,10.88 S7.1 53.12,11.25 v53.12,18.75 | S10.1 62.75,63.12 62.75,61.12 64.25,59.62 64.25,42.12 62.75,40.62 S13.1 62.62,40.25 60.5,40.25 60.38,40.12 R29.2 60,40 56.62,40 D5.A
  Bottom 0.61: v53.12,18.75 62.88,28.5 62.88,35.86 60.38,38.36 60.38,40 R29.2
PB0  (via drill 0.65 pad 1.3)
  Top 0.61: IC4.14 36.75,36.25 35.62,37.38 35.62,37.5 34.62,38.5 22.51,38.5 20.62,40.26 10.16,40.26 7.48,42.94 v7.48,56.65
  Bottom 0.61: v7.48,56.65 5.08,59.7 5.08,65.41 5.58,65.95 12,72.38 SV1.1
PB1  (via drill 0.61 pad 1.3)
  Top 0.61: v21.37,36.76 21.37,36.28 23.5,34.16 23.5,34.12 37.38,34.12 39.38,36.12 IC4.15
  Bottom 0.61: v21.37,36.76 21.37,37.63 21.59,37.85 21.5,44 19.78,45.72 15.88,45.72 13.84,47.75 13.97,53.41 8.6,58.79 8.6,67.52 10.79,69.85 12.83,69.85 14.5,71.52 14.5,72.38 SV1.2
PC0  (via drill 0.61 pad 1.3)
  Top 0.61: v40.25,51.88 39.56,51.88 37.59,53.85 37.5,54.5 IC2.11 | v12.36,25.62 25.13,25.62 27.94,28.32 28,28.38 28,29.12 IC3.11 | v14.48,42.85 12.4,42.85 10.62,44.63 10.49,64.13 10.5,64.62 10.5,66.25 11.62,67.38 17.97,67.38 20.7,70.1 31.5,70.1 32.38,70.99 SV1.9
  Bottom 0.61: IC3.11 28,29.12 29.12,28 29.12,27.88 29.88,27.12 46.25,27.12 48.25,29.12 IC1.11 48.25,29.5 48.25,37.75 47.38,38.62 47.37,47.12 48.01,47.88 48.01,49.4 47.24,50.29 46.58,50.29 45.25,51.63 45,51.63 45,51.62 40.45,51.62 40.39,51.69 v40.25,51.88 | v14.48,42.85 14.86,42.8 15.88,41.78 15.88,38.1 13.34,35.56 13.34,33.4 13.21,33.27 10.75,30.89 10.75,27.36 v12.36,25.62
PC1  (via drill 0.61 pad 1.3)
  Top 0.61: v53.75,67.33 v53.75,67.34 53.75,57.99 55.25,56.49 55.25,48.35 50.12,43.23 50.12,39.62 49.38,38.88 49.38,38.33 46.99,35.94 46.99,34.92 45.09,33.02 42.55,33.02 40.64,31.11 IC1.14 | v51.25,70.25 51.4,70.25 48.62,67.48 43.41,67.48 40.89,70 35.92,70 34.92,70.99 SV1.10
  Bottom 0.61: v53.75,67.33 53.75,67.79 53.72,67.82 51.75,69.88 v51.25,70.25
PC2  (via drill 0.61 pad 1.3)
  Top 0.61: v56.5,56.76 56.52,56.01 56.5,47.53 51.25,42.28 51.25,39 50.8,38.55 50.8,38.1 48.26,35.56 48.26,34.29 45.62,31.66 45.62,29.25 IC1.12 | v13.36,27.12 23.5,27.12 25.5,29.12 IC3.12
  Bottom 0.61: 25.5,29.25 IC3.12 25.4,30.35 27.18,32.13 42.87,32.13 45.75,29.25 IC1.12 | v56.5,56.76 55.49,56.76 54.25,58 40.26,58.04 39.75,58.42 38.1,58.42 38.1,58.35 35,55.25 35,54.62 IC2.12 | v13.36,27.12 13.38,27.12 11.88,28.62 11.88,30.39 14.48,33.02 14.48,35.18 17.09,37.79 17.12,37.79 17,42.97 12.21,47.62 7.62,47.62 3.81,51.44 3.83,57.78 3.83,66.83 10.87,74.5 35.5,74.5 36.25,73.75 36.25,73.62 37.38,72.5 SV1.11
PC3  (via drill 0.61 pad 1.3, 0.65 pad 1.3)
  Top 0.61: 14.61,34.29 17.78,34.29 22.75,29.5 22.75,29.25 IC3.13 | 5.71,53.77 5.71,68.72 10.87,74.5 38.91,74.5 40.13,73.28 40,72.5 SV1.12 | v54.6,7.23 55.24,7.23 57.62,9.62 57.62,12 57,12.62 57,23.52 55.77,24.88 47.38,24.88 44.38,27.88 44.38,28 43.25,29.12 IC1.13 | v9.88,14.62 9.91,29.84 8.48,31.27 8.48,32.75 10.02,34.29 10.03,34.29 | 14.69,34.39 14.61,34.29 | 10.03,34.29 14.61,34.29 | v17.48,61.5 16.93,61.5 15.24,59.69 15.24,55.99 v12.5,51.73 | v5.72,51.73 5.71,53.77 | 5.71,53.77 5.71,46.99 5.72,46.91 5.72,40.25 10.03,35.69 10.03,34.29
  Bottom 0.61: v54.6,7.23 54.6,7.25 53.72,8.13 16.12,8.38 v9.88,14.62 | IC2.13 32.38,54.62 31.25,55.75 31.25,55.88 28.25,58.88 21.25,58.88 18.62,61.5 v17.48,61.5 | v12.5,51.73 v5.72,51.73
PC4  (via drill 0.61 pad 1.3)
  Top 0.61: v65.63,57.26 65.63,70.75 61.75,74.5 43.64,74.5 42.55,73.41 42.5,72.5 SV1.13
  Bottom 0.61: v65.63,57.26 65.5,57.24 65.41,57.15 60.33,57.15 59.8,56.62 59.75,56.62 58.25,55.12 52.75,55.12 R26.1
PC5  (via drill 0.61 pad 1.3)
  Top 0.61: v56,63.49 56,58.5 R27.1
  Bottom 0.61: v56,63.49 57.66,65.28 57.66,66.29 58.8,67.44 59.31,67.44 61.75,69.88 61.75,73.62 60.88,74.5 46.18,74.5 45.09,73.41 45.12,72.5 SV1.14
PC6
  Bottom 0.61: SV1.15 47.62,71.75 46.35,70.48 R28.1
PC7  (via drill 0.61 pad 1.3)
  Top 0.61: R29.1 52.75,40.12 52.83,40.12 52.83,41.78 59.44,48.39 60.21,48.39 v60.23,48.41 | SV1.16 50.16,71.5 48.66,70 v48.12,70
  Bottom 0.61: 48.38,70 v48.12,70 48.12,69.73 50.29,67.56 51.18,67.56 53.21,65.53 53.21,64.52 54.36,63.37 54.36,62.87 55.37,61.85 58.76,61.85 59.79,62.88 63.75,62.88 66.17,60.45 69.85,60.45 70.64,59.66 70.64,55.26 63.41,48.66 60.48,48.66 v60.23,48.41
PD7  (via drill 0.61 pad 1.3)
  Top 0.61: v52,63.1 52,64.19 52.58,64.77 52.58,66.17 51.82,66.93 51.82,67.69 52.62,68.5 52.62,72.38 SV1.17
  Bottom 0.61: v52,63.1 50.48,63.1 49,61.62 R25.1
